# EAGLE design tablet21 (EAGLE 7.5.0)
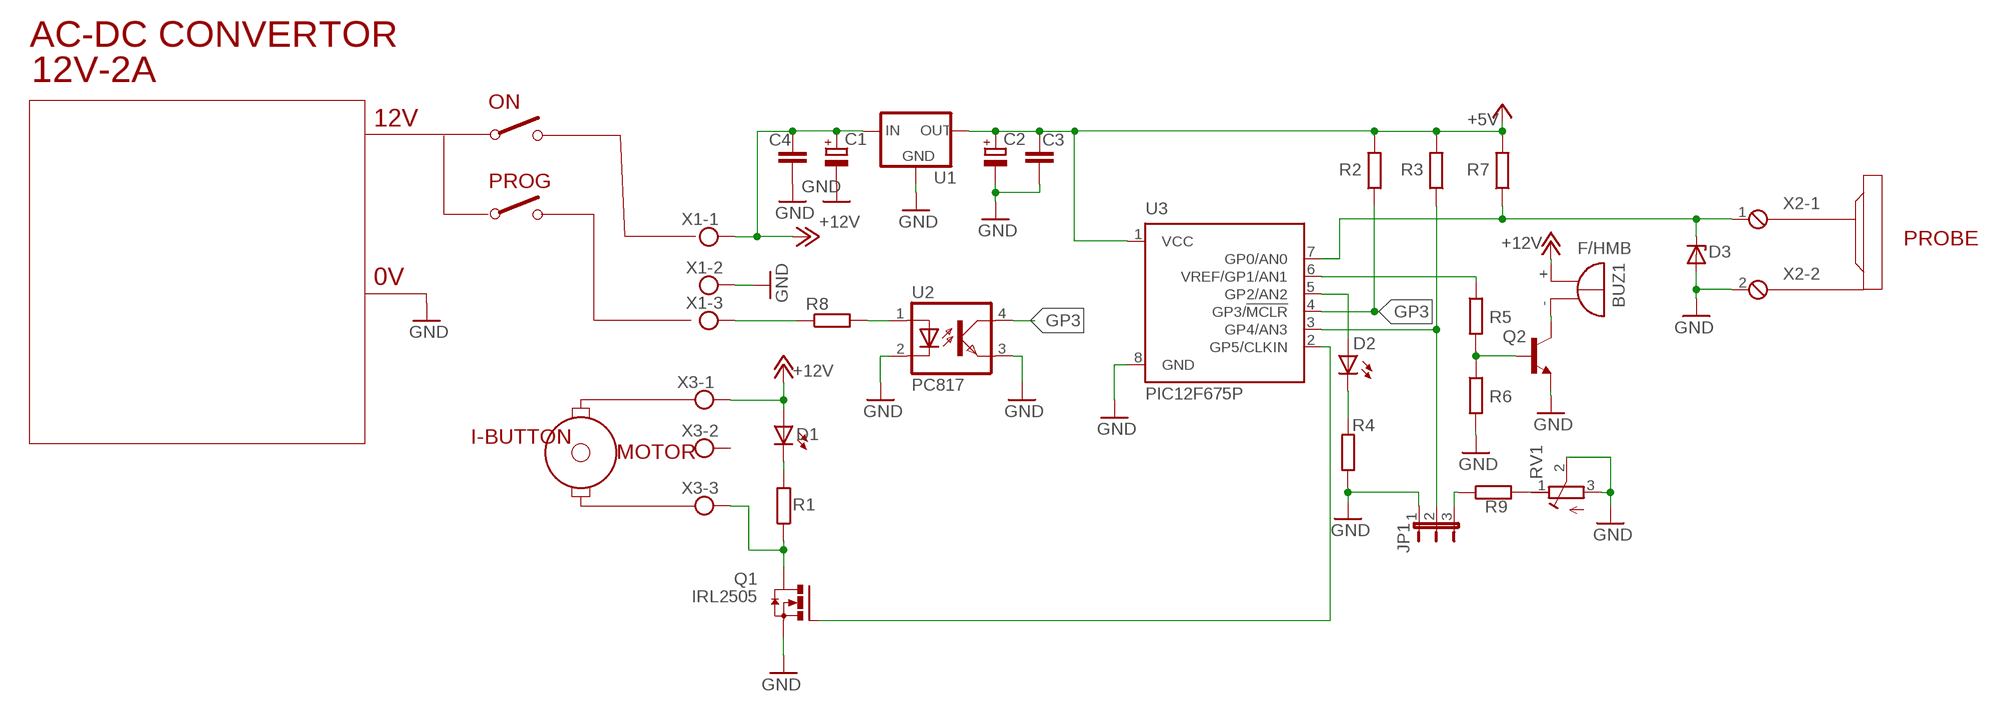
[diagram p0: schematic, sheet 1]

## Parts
BUZ1  F/HMB  [F/HMB]
C1  CPOL-EUE2-4  [E2-4]
C2  CPOL-EUE2-4  [E2-4]
C3  C-EUC1206  [C1206]
C4  C-EUC1206  [C1206]
D1  LED3MM  [LED3MM]
D2  LED3MM  [LED3MM]
D3  ZENER-DIODEDO35Z10  [DO35Z10]
JP1  JP2E  [JP2]
Q1  IRL2505  IRF3704-H  [TO220BH]
Q2  BC337  [TO92]
R1  R-EU_R1206  [R1206]
R2  R-EU_R1206  [R1206]
R3  R-EU_R1206  [R1206]
R4  R-EU_R1206  [R1206]
R5  R-EU_R1206  [R1206]
R6  R-EU_R1206  [R1206]
R7  R-EU_R1206  [R1206]
R8  R-EU_R1206  [R1206]
R9  R-EU_R1206  [R1206]
RV1  R-TRIMM-3386-F  [R-TRIMM-3386F]
U1  78LXX  [78LXX]
U2  PC817  [DIL04]
U3  PIC12F675P  [DIL8]
X1  MKDSN1,5/3-5,08  [MKDSN1,5/3-5,08]
X2  MPT2  [2POL254]
X3  MKDSN1,5/3-5,08  [MKDSN1,5/3-5,08]

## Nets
+5V: C2.+ C3.1 R2.2 R3.2 R7.2 U1.OUT U3.1(VCC)
+12V: BUZ1.+ C1.+ C4.1 D1.A U1.IN X1.1 X3.1
GND: C1.- C2.- C3.2 C4.2 D3.A JP1.1 Q1.S Q2.1(E) R4.1 R6.2 RV1.2(S) RV1.3(E) U1.GND U2.2(C) U2.3(EMIT) U3.8(GND) X1.2 X2.2
GP3: R2.1 U2.4(COL) U3.4(GP3/!MCLR)
N$1: Q1.G U3.2(GP5/CLKIN)
N$2: R8.2 U2.1(A)
N$3: D2.K(C) R4.2
N$4: R8.1 X1.3
N$5: R9.2 RV1.1(A)
N$6: Q1.D R1.1 X3.3
N$7: D1.K(C) R1.2
N$8: JP1.2 R3.1 U3.3(GP4/AN3)
N$9: JP1.3 R9.1
N$10: D2.A U3.5(GP2/AN2)
N$11: R5.1 U3.6(VREF/GP1/AN1)
N$12: Q2.2(B) R5.2 R6.1
N$13: BUZ1.- Q2.3(C)
N$14: D3.C R7.1 U3.7(GP0/AN0) X2.1
Unconnected: X3.2

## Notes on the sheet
- AC-DC CONVERTOR
- 12V-2A
- ON
- 12V
- PROG
- PROBE
- 0V
- I-BUTTON | MOTOR

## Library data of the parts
BUZ1 = buzzer:F/HMB: BUZZER; OC_FARNELL: unknown; OC_NEWARK: unknown
C1 C2 = rcl:CPOL-EU: POLARIZED CAPACITOR, European symbol
C3 C4 = rcl:C-EU: CAPACITOR, European symbol
D1 D2 = led:LED: LED
D3 = diode:ZENER-DIODE: Z-Diode
JP1 = jumper:JP2E: JUMPER
Q1 = transistor-power:IRF3704: SMPS MOSFET HEXFET® Power MOSFET Source: http://www.irf.com/product-info/datasheets/data/irf3704.pdf
Q2 = transistor:BC337: NPN TRANSISTOR
R1-R9 = rcl:R-EU_: RESISTOR, European symbol
RV1 = rcl:R-TRIMM-3386-F
U1 = v-reg:78LXX: VOLTAGE REGULATOR
U2 = optocoupler:PC817: SHARP OPTO COUPLER; MPN: PC817X4J000F; OC_FARNELL: 9707727; OC_NEWARK: 97K7059
U3 = microchip:PIC12F675: 8-Pin FLASH-Based 8-Bit CMOS Microcontroller Precision Internal 4 MHz oscillator factory calibrated to ±1% Low Power Features: Standby Current: - 1 nA @ 2.0V, typical Operating Current: - 8.5&micro;A @ 32 kHz, 2.0V, typical - 100&micro;A @ 1 MHz, 2.0V, typical Watchdog Timer Current: - 300 nA @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; MF: MICROCHIP; MPN: PIC12F675-E/P; OC_FARNELL: 9759018; OC_NEWARK: 92C4340
X1 X3 = con-phoenix-508:MKDSN1,5/3-5,08: MKDSN 1,5/ 3-5,08 Printklemme Nennstrom: 13,5 A Nennspannung: 250 V Rastermaß: 5,08 mm Polzahl: 3 Anschlussart: Schraubanschluss Montage: Löten Anschlussrichtung Leiter/Platine: 0 ° Artikelnummer: 1729131 Source: http://eshop.phoenixcontact.com .. 1729131.pdf
X2 = con-phoenix-254:MPT2: PHOENIX CONNECTOR; OC_FARNELL: unknown; OC_NEWARK: unknown

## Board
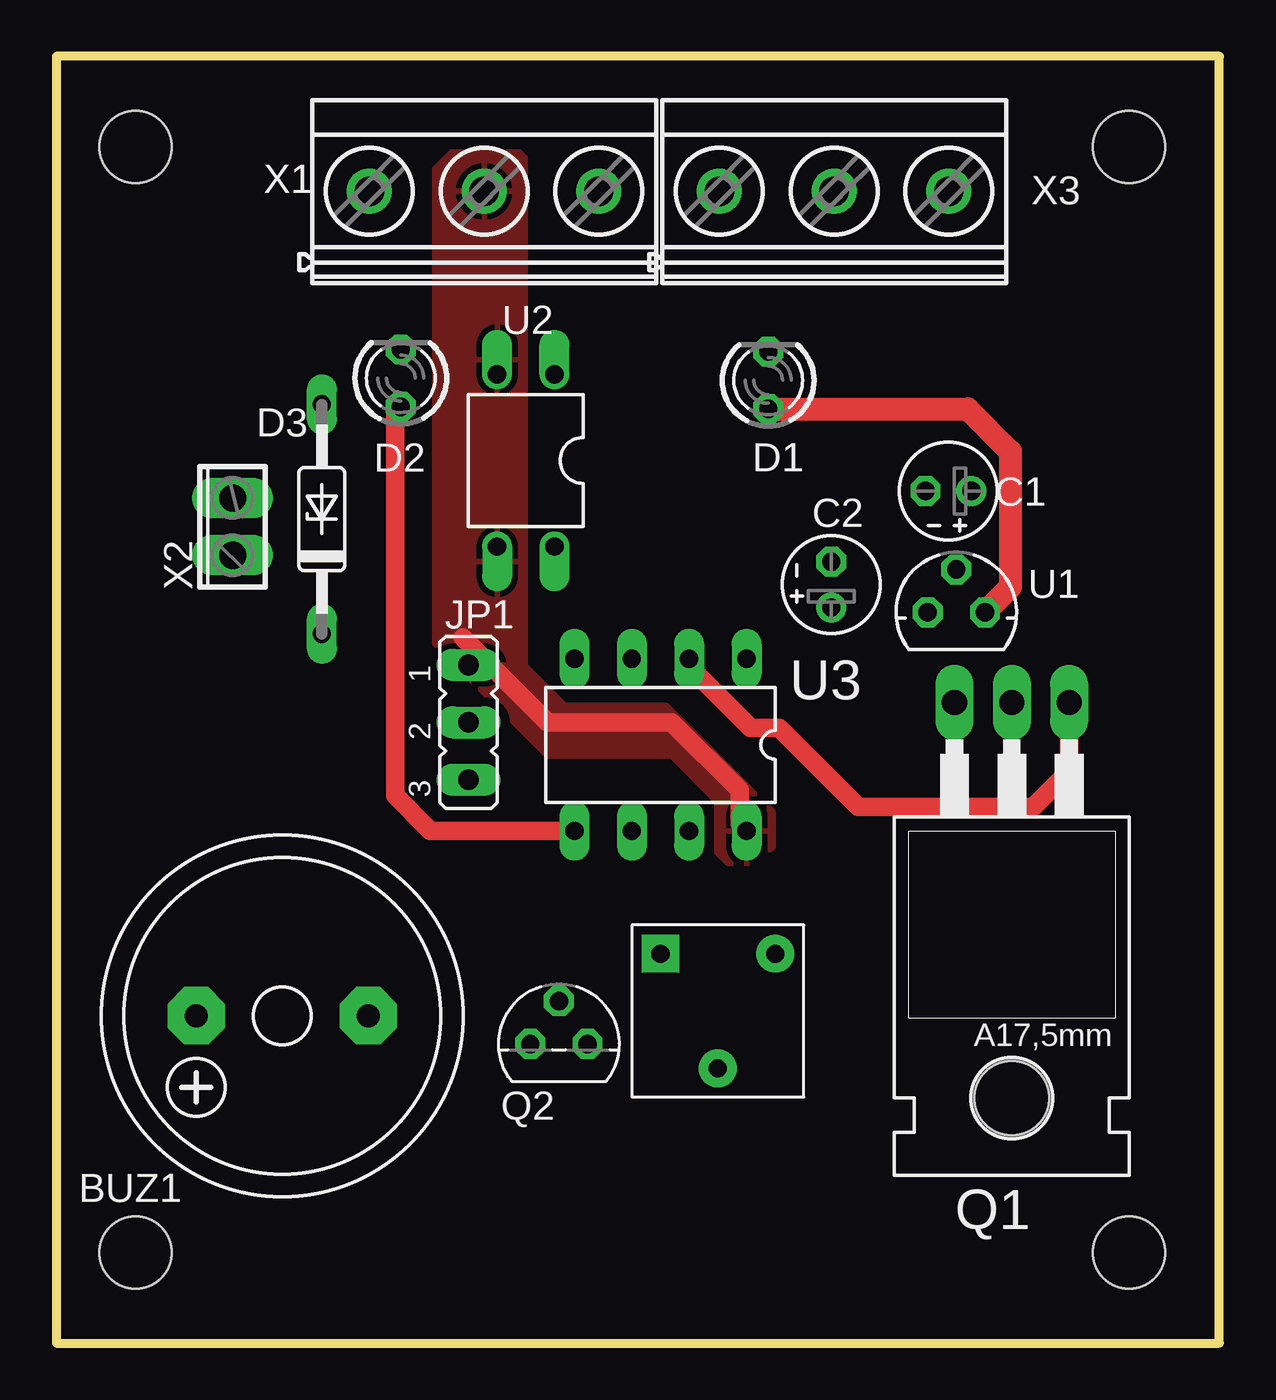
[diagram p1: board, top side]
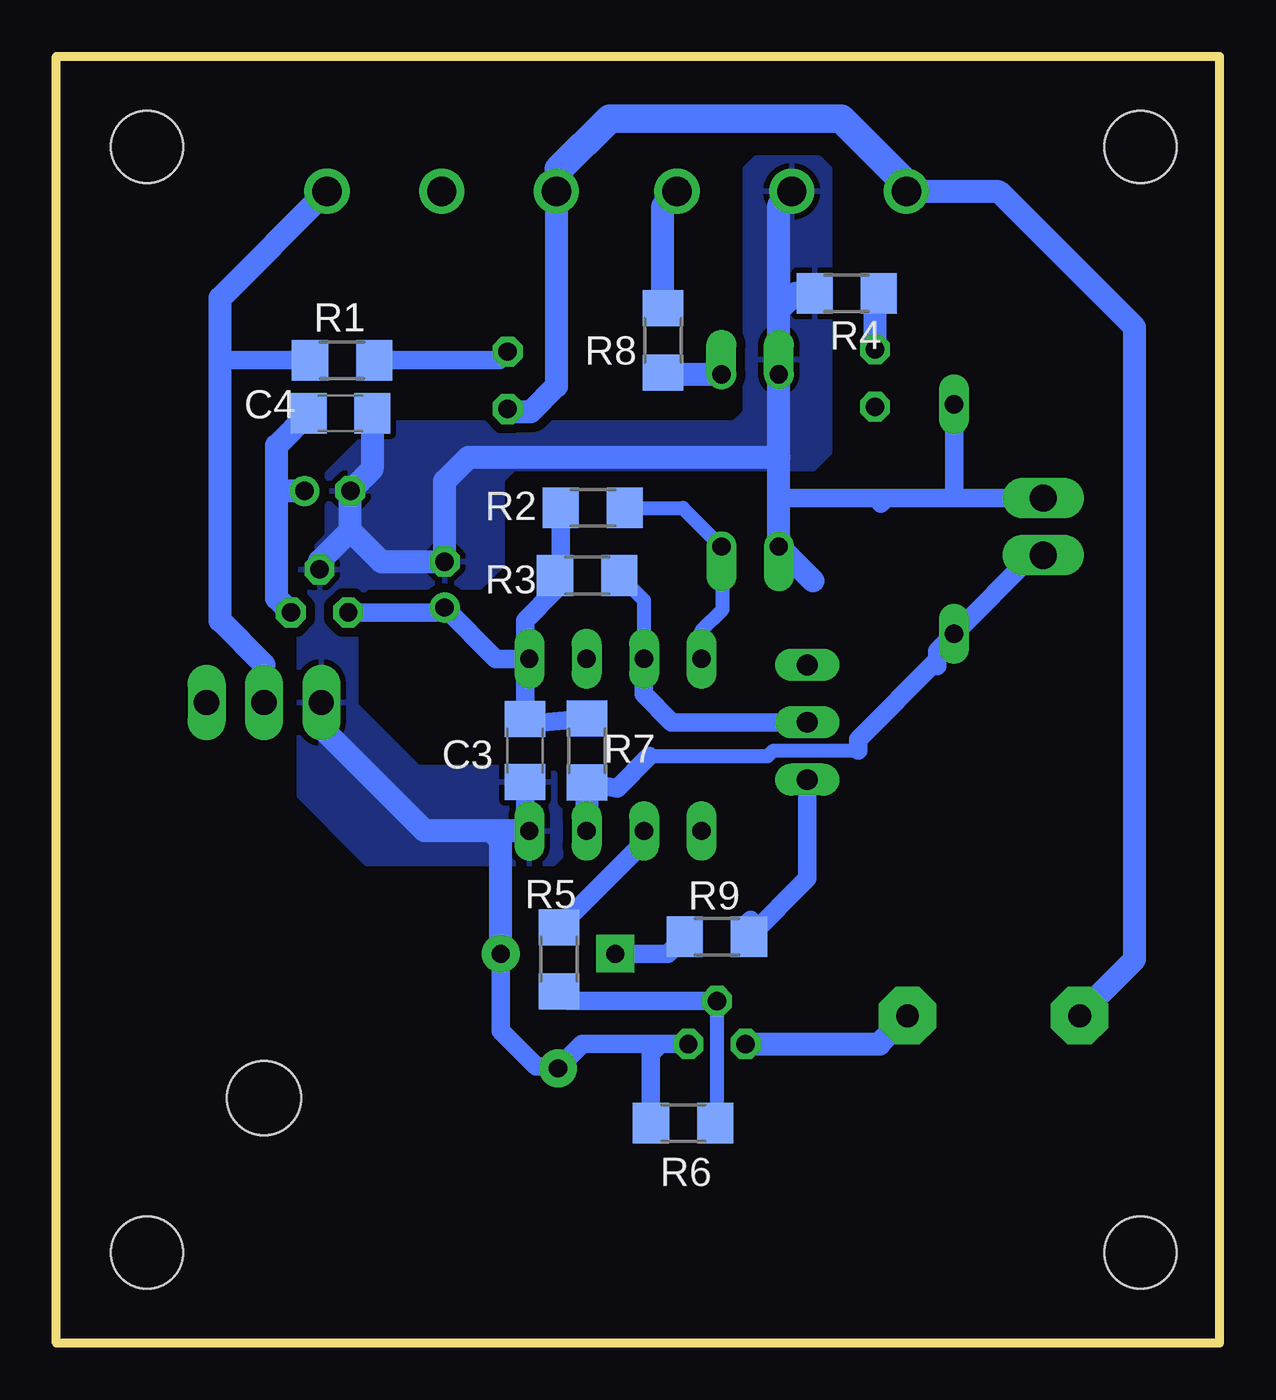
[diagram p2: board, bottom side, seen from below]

Size 51.5 x 57 mm. Coordinates in mm from the lower left corner, seen from the top.
Outline: 0,0 51.5,0 51.5,57 0,57 0,0
Copper layers (1*16): Top 0.035mm / dielectric 1.5mm / Bottom 0.035mm
Design rules "default": minimum track width 10mil, minimum drill 24mil, track to track 8mil, track to pad 8mil, pad to pad 8mil, via to via 8mil, smd to smd 8mil, copper to edge 40mil, drill to drill 8mil, minimum pad ring 10mil, minimum via ring 8mil, stop-mask expansion 4mil, vias tented up to drill 0mil, thermal gap 10mil
Holes 3.2 mm at 3.5,4 3.5,53 47.5,53 47.5,4

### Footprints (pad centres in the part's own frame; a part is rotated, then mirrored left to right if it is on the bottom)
F/HMB = drill 1.016 pad 2.54 octagon: + 3.81,0; - -3.81,0
E2-4 = drill 0.813 pad 1.27: + -1.016,0 | drill 0.813 pad 1.27 octagon: - 1.016,0
C1206 = smd 1.6 x 1.8: 1 -1.4,0; 2 1.4,0
LED3MM = drill 0.813 octagon: A -1.27,0; K 1.27,0
DO35Z10 = drill 0.813 long: A 5.08,0; C -5.08,0
JP2 = drill 0.914 long: 1 -2.54,0; 2 0,0; 3 2.54,0
TO220BH = drill 1.118 long: D 0,-6.35; G -2.54,-6.35; S 2.54,-6.35 | hole 3.302: 0,11.176
TO92 = drill 0.813 octagon: 1 1.27,0; 2 0,1.905; 3 -1.27,0
R1206 = smd 1.6 x 1.803: 1 -1.422,0; 2 1.422,0
R-TRIMM-3386F = drill 0.8 pad 1.676 square: 1 0,0 | drill 0.8 pad 1.676: 2 5.08,2.54; 3 0,5.08
78LXX = drill 0.813 octagon: GND 0,1.905; IN 1.27,0; OUT -1.27,0
DIL04 = drill 0.813 offset: 1 -1.27,-3.81; 2 1.27,-3.81; 3 1.27,3.81; 4 -1.27,3.81
DIL8 = drill 0.813 long: 1 -3.81,-3.81; 2 -1.27,-3.81; 3 1.27,-3.81; 4 3.81,-3.81; 5 3.81,3.81; 6 1.27,3.81; 7 -1.27,3.81; 8 -3.81,3.81
MKDSN1,5/3-5,08 = drill 1.3 pad 2: 1 -7.641,0.025; 2 -2.561,0.025; 3 2.519,0.025
2POL254 = drill 1.2 long: 1 -1.27,0; 2 1.27,0

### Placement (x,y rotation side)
BUZ1  10,14.5 180 top
C1  39.5,37.75 180 top
C2  34.31,33.6 90 top
C3  30.75,26.25 270 bottom
C4  38.92,41.19 0 bottom
D1  31.52,42.65 90 top
D2  15.25,42.75 90 top
D3  11.75,36.5 90 top
JP1  18.25,27.5 270 top
Q1  42.31,22.03 180 top
Q2  22.25,13.25 0 top
R1  38.85,43.54 0 bottom
R2  27.75,37 180 bottom
R3  28,34 180 bottom
R4  16.5,46.5 0 bottom
R5  29.25,17 270 bottom
R6  23.75,9.75 180 bottom
R7  28,26.25 90 bottom
R8  24.64,44.42 270 bottom
R9  22.25,18 180 bottom
RV1  26.75,17.25 270 top
U1  39.85,32.37 0 top
U2  20.78,39.1 180 top
U3  26.75,26.5 180 top
X1  21.5,51 0 top
X2  7.8,36.17 90 top
X3  37,51 0 top

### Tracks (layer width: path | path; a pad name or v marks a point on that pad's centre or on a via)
+5V
  Bottom 0.813: U1.OUT 34.52,32.37 C2.+ 32.04,30.31 U3.1 | U3.1 30.75,30.12 C3.1 30.73,27.42 R7.2 | R2.2 29.17,34.25 R3.2 29.42,33.33 30.75,32 30.75,30.5 U3.1
+12V
  Top 1.016: D1.A 40.37,41.38 42.25,39.5 42.25,33.5 U1.IN
  Bottom 1.016: U1.IN 41.75,33 41.75,38 | 41.75,38 41.75,39.76 C4.1 | BUZ1.+ 6.19,14.56 3.75,17 3.75,45 9.75,51 13.83,51 X1.1 | C1.+ 41.5,37.75 41.75,38 | X3.1 29.36,42.39 30.5,41.25 31.39,41.25 D1.A
  Bottom 1.27: X1.1 13.86,51.36 16.75,54.25 27,54.25 29.25,52 29.25,51.13 X3.1
GND
  Top 0.813: 18,31.25 21.75,27.5 27.25,27.5 30.25,24.5 30.25,23 U3.8
  Bottom 0.813: Q2.1 24.75,13.25 | 24.75,13.25 28.21,13.25 RV1.2 29.37,12.25 30.25,12.25 31.83,13.83 RV1.3 | R6.2 25.17,12.83 24.75,13.25 | C3.2 30.75,22.88 U3.8 | X2.2 11.5,37.44 | 11.5,37.44 14.75,37.44 | 14.75,37.44 19.32,37.44 19.51,37.25 | 11.5,37.44 11.75,37.69 D3.A | 15,37.19 14.75,37.44
  Bottom 1.016: U3.8 32.25,22.69 | 32.25,22.69 35.19,22.69 39.75,27.25 39.75,28.36 Q1.S | U1.GND 39.85,34.65 38.5,36 | 38.5,36 38.5,37.73 C1.- 37.52,38.71 C4.2 | 38.5,36 37.12,34.62 C2.- 34.31,38.19 33.25,39.25 19.51,39.25 | 18,33.78 U2.3 19.51,37.25 19.51,39.25 | 19.51,39.25 U2.2 19.51,45.75 | 19.51,45.75 19.51,50.45 X1.2 | RV1.3 31.83,22.27 32.25,22.69 | R4.1 18.76,46.5 19.51,45.75
  pour Bottom (isolate 0.406): 30,25.5 35.5,25.5 38.25,28.25 38.25,33 37.75,33.5 32.75,33.5 31.75,34.5 31.75,38.25 31.25,38.75 18,38.75 17.25,39.5 17.25,52 17.75,52.5 20.5,52.5 21,52 21,41.25 21.5,40.75 37.25,40.75 39.5,38.5 39.5,35.75 40.75,34.5 40.75,24.25 38,21.5 37.75,21.25 29.5,21.25 29,21.75 29,24.75 29.75,25.5
  pour Top (isolate 0.406): 31,21.25 31.75,22 31.75,23.5 27,28.25 22.5,28.25 20.75,30 20.75,52.5 20.5,52.75 17.5,52.75 17.25,52.5 16.75,52 16.75,31 21.75,26 27.25,26 29.25,24 29.25,21.75 29.75,21.25
GP3
  Bottom 0.61: U3.4 22.94,31.56 22,32.5 22,35.24 U2.4 23.76,37 R2.1
N$1
  Top 0.813: Q1.G 44.85,25.35 43.25,23.75 35.5,23.75 32,27.25 30.75,27.25 28.25,29.75 28.25,30.08 U3.2
N$2
  Bottom 1.016: U2.1 24.55,42.91 R8.2
N$3
  Bottom 1.016: D2.K 15.25,46.33 R4.2
N$4
  Bottom 1.016: R8.1 24.64,50.4 X1.3
N$5
  Bottom 0.813: RV1.1 24.42,17.25 R9.2
N$6
  Bottom 0.813: R1.1 43.96,43.54 44.25,43.25
  Bottom 1.016: Q1.D 42.31,30.06 44.25,32 44.25,43.25 44.25,46.29 X3.3
N$7
  Bottom 0.813: R1.2 31.9,43.54 D1.K
N$8
  Bottom 0.61: U3.3 25.48,32.9 R3.1
  Bottom 0.813: JP1.2 24.25,27.5 25.5,28.75 25.5,30.29 U3.3
N$9
  Bottom 0.813: 20.75,18.75 21,18.5 21,18.17 R9.1 18.25,20.58 JP1.3
N$10
  Top 0.813: D2.A 15,41.23 15,24.25 16.56,22.69 U3.5
N$11
  Bottom 0.813: U3.6 25.48,22.19 R5.1
N$12
  Bottom 0.61: Q2.2 22.25,9.83 R6.1
  Bottom 0.813: Q2.2 28.83,15.15 R5.2
N$13
  Bottom 1.016: Q2.3 15.06,13.25 BUZ1.-
N$14
  Bottom 0.61: 28.02,24.56 R7.1 | 25.25,26 20,26 19.75,26.25 16,26.25
  Bottom 0.813: R7.1 26.67,24.58 25.25,26 | X2.1 8.27,34.9 D3.C 12.5,30.67 12.5,30.25 | 12.5,30 12.5,30.25 | 16,26.25 16,26.75 12.5,30.25
  Bottom 1.016: 28.02,24.56 U3.7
